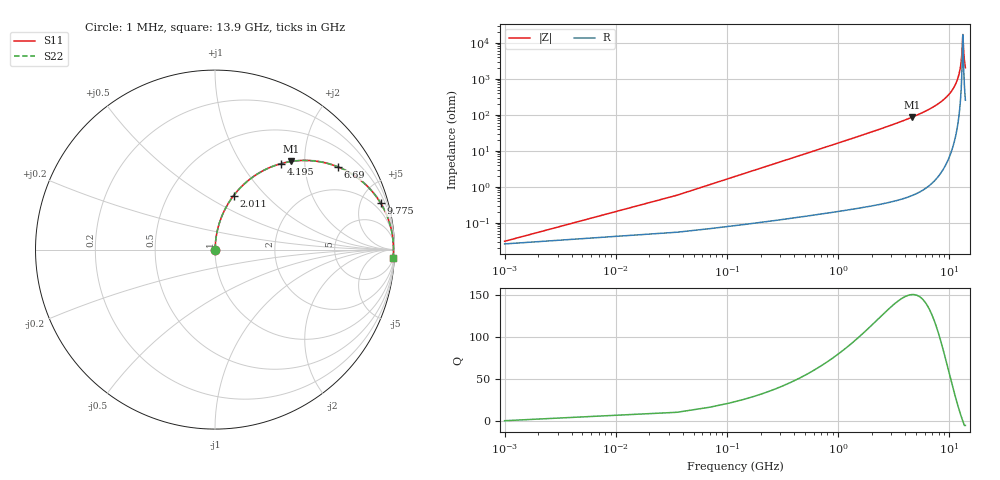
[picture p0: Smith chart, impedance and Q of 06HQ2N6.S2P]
! Coilcraft 0604HQ-2N6 Chip Inductor
! 15 August 2002
# MHZ S MA R 50
!Freq  MagS11  AngS11  MagS21  AngS21  MagS12  AngS12  MagS22  AngS22
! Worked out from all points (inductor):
!   403 points, 1 MHz to 13.9 GHz, reference 50 ohm
!   read as one part in series: L = 2.6 nH near 70.32 MHz
!   highest Q = 150 at 4.611 GHz (marker M1), where L = 2.96 nH
!   self-resonance near 13.17 GHz
!   S11 on the Smith chart (normalised r, x): 1 MHz: 1.00, +0.00; 2.011 GHz: 1.01, +0.67; 4.195 GHz: 1.01, +1.52; 6.69 GHz: 1.02, +2.94; 9.775 GHz: 1.12, +7.08; 13.9 GHz: 6, -40
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1  0.0003054 32.3  0.9997 -0.0  0.9997 -0.0  0.0003054 32.3
104.98  0.01715 86.4  0.9991 -1.0  0.9991 -1.0  0.01715 86.4
208.96  0.03411 86.3  0.9984 -2.0  0.9984 -2.0  0.03411 86.3
347.6  0.05667 85.5  0.9971 -3.2  0.9971 -3.2  0.05667 85.5
936.82  0.1517 80.5  0.9865 -8.7  0.9865 -8.7  0.1517 80.5
2011.28  0.318 71.0  0.9453 -18.5  0.9453 -18.5  0.318 71.0
2323.22  0.3637 68.2  0.9285 -21.3  0.9285 -21.3  0.3637 68.2
4194.86  0.6043 52.4  0.7927 -37.2  0.7927 -37.2  0.6043 52.4
4610.78  0.6491 49.1  0.7564 -40.5  0.7564 -40.5  0.6491 49.1
4645.44  0.6527 48.9  0.7533 -40.7  0.7533 -40.7  0.6527 48.9
6690.38  0.8242 34.1  0.5601 -55.5  0.5601 -55.5  0.8242 34.1
6967.66  0.8418 32.2  0.5332 -57.3  0.5332 -57.3  0.8418 32.2
9289.88  0.9451 18.3  0.3139 -70.9  0.3139 -70.9  0.9451 18.3
9775.12  0.9583 15.7  0.2705 -73.4  0.2705 -73.4  0.9583 15.7
11612.1  0.9881 6.7  0.1173 -80.8  0.1173 -80.8  0.9881 6.7
12235.98  0.9923 4.0  0.06943 -81.7  0.06943 -81.7  0.9923 4.0
12651.9  0.9938 2.2  0.03884 -79.7  0.03884 -79.7  0.9938 2.2
12894.52  0.9942 1.2  0.02166 -73.9  0.02166 -73.9  0.9942 1.2
13171.8  0.9943 0.1  0.005849 -12.7  0.005849 -12.7  0.9943 0.1
13241.12  0.9943 -0.2  0.006744 31.5  0.006744 31.5  0.9943 -0.2
13553.06  0.9938 -1.4  0.02571 75.3  0.02571 75.3  0.9938 -1.4
13900  0.9928 -2.8  0.04868 80.1  0.04868 80.1  0.9928 -2.8
